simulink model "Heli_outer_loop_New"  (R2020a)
settings: Solver=FixedStepDiscrete  StartTime=0.0  StopTime=10.0  FixedStep=0.01  RelTol=1e-3  EnableMultiTasking=on
model workspace (MAT data in the model file):
  Ts : Simulink.Parameter (value not decoded)
symbols that are objects in the model workspace (value not decoded): Ts
undefined symbols (not defined in the file or in its folder): DiscIntNeverNeededParam
libraries: simulink x1

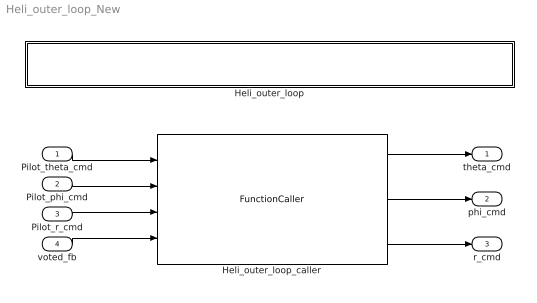
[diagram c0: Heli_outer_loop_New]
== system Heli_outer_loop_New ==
  Pilot_theta_cmd : Inport
  Pilot_phi_cmd : Inport  Port=2
  Pilot_r_cmd : Inport  Port=3
  voted_fb : Inport  Port=4
  Heli_outer_loop : Subsystem  TreatAsAtomicUnit=on
  Heli_outer_loop_caller : FunctionCaller  FunctionPrototype=[theta_cmd,phi_cmd,r_cmd] = Heli_outer_loop(Pilot_theta_cmd,Pilot_phi_cmd,Pilot_r_cmd,voted_fb)
  theta_cmd : Outport
  phi_cmd : Outport  Port=2
  r_cmd : Outport  Port=3
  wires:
  Pilot_theta_cmd/1 -> Heli_outer_loop_caller/1
  Pilot_phi_cmd/1 -> Heli_outer_loop_caller/2
  Pilot_r_cmd/1 -> Heli_outer_loop_caller/3
  voted_fb/1 -> Heli_outer_loop_caller/4
  Heli_outer_loop_caller/1 -> theta_cmd/1
  Heli_outer_loop_caller/2 -> phi_cmd/1
  Heli_outer_loop_caller/3 -> r_cmd/1

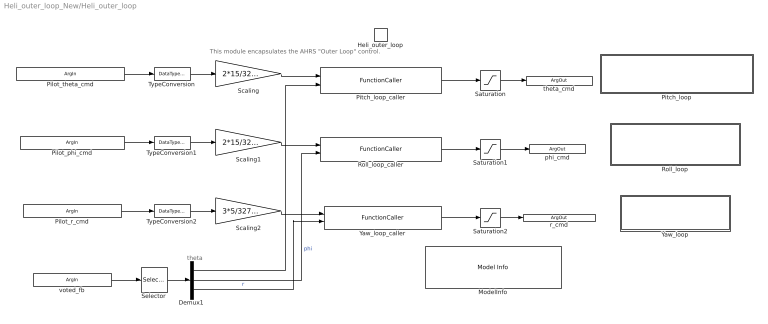
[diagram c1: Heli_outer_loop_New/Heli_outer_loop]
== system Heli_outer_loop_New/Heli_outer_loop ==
  note: theta
  note: This module encapsulates the AHRS "Outer Loop" control.
  Heli_outer_loop : TriggerPort  TriggerType=function-call  IsSimulinkFunction=on  FunctionName=Heli_outer_loop  FunctionVisibility=scoped  VariantControl=Variant  PortDimensions=1
  Demux1 : Demux  Outputs=3
  ModelInfo : simulink/Model-Wide Utilities/Model Info  Frame=on  DisplayStringWithTags=|  HorizontalTextAlignment=Center  LeftAlignmentValue=0.5
      | Model Name: %<ModelName>
      | Model Version: %<ModelVersion>
      | Last Modified: %<LastModificationDate>
      | 
      | Copyright 2016 The MathWorks, Inc.
  Pitch_loop : Subsystem  TreatAsAtomicUnit=on
  Pitch_loop_caller : FunctionCaller  FunctionPrototype=theta_cmd = Pitch_loop(Pilot_theta_cmd,theta)  InputArgumentSpecifications=double(1),double(1)  OutputArgumentSpecifications=double(1)
  Roll_loop : Subsystem  TreatAsAtomicUnit=on
  Roll_loop_caller : FunctionCaller  FunctionPrototype=phi_cmd = Roll_loop(Pilot_phi_cmd,phi)  InputArgumentSpecifications=double(1),double(1)  OutputArgumentSpecifications=double(1)
  Saturation : Saturate  UpperLimit=30  LowerLimit=-30
  Saturation1 : Saturate  UpperLimit=30  LowerLimit=-30
  Saturation2 : Saturate  UpperLimit=30  LowerLimit=-30
  Scaling : Gain  Gain=2*15/32767
  Scaling1 : Gain  Gain=2*15/32767
  Scaling2 : Gain  Gain=3*5/32767
  Selector : Selector  InputPortWidth=5  IndexOptions=Index vector (dialog)  Indices=[1 2 3]  OutputSizes=1
  TypeConversion : DataTypeConversion  OutDataTypeStr=double
  TypeConversion1 : DataTypeConversion  OutDataTypeStr=double
  TypeConversion2 : DataTypeConversion  OutDataTypeStr=double
  Yaw_loop : Subsystem  TreatAsAtomicUnit=on
  Yaw_loop_caller : FunctionCaller  FunctionPrototype=r_cmd = Yaw_loop(Pilot_r_cmd,r)  InputArgumentSpecifications=double(1), double(1)  OutputArgumentSpecifications=double(1)
  Pilot_theta_cmd : ArgIn  OutDataTypeStr=int16  ArgumentName=Pilot_theta_cmd
  Pilot_phi_cmd : ArgIn  Port=2  OutDataTypeStr=int16  ArgumentName=Pilot_phi_cmd
  Pilot_r_cmd : ArgIn  Port=3  OutDataTypeStr=int16  ArgumentName=Pilot_r_cmd
  voted_fb : ArgIn  Port=4  PortDimensions=5  ArgumentName=voted_fb
  theta_cmd : ArgOut  ArgumentName=theta_cmd
  phi_cmd : ArgOut  Port=2  ArgumentName=phi_cmd
  r_cmd : ArgOut  Port=3  ArgumentName=r_cmd
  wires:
  Selector/1 -> Demux1/1
  TypeConversion2/1 -> Scaling2/1
  Pilot_r_cmd/1 -> TypeConversion2/1
  Pilot_phi_cmd/1 -> TypeConversion1/1
  Saturation1/1 -> phi_cmd/1
  TypeConversion1/1 -> Scaling1/1
  Saturation2/1 -> r_cmd/1
  voted_fb/1 -> Selector/1
  Roll_loop_caller/1 -> Saturation1/1
  Yaw_loop_caller/1 -> Saturation2/1
  TypeConversion/1 -> Scaling/1
  Saturation/1 -> theta_cmd/1
  Pilot_theta_cmd/1 -> TypeConversion/1
  Scaling/1 -> Pitch_loop_caller/1
  Demux1/1 -> Pitch_loop_caller/2
  Scaling1/1 -> Roll_loop_caller/1
  Demux1/2 -> Roll_loop_caller/2  "phi"
  Pitch_loop_caller/1 -> Saturation/1
  Scaling2/1 -> Yaw_loop_caller/1
  Demux1/3 -> Yaw_loop_caller/2  "r"

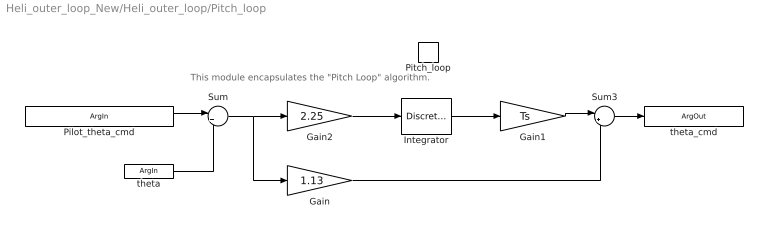
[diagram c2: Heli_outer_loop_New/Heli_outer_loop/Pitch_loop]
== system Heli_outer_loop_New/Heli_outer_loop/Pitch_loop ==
  note: This module encapsulates the "Pitch Loop" algorithm.
  Pitch_loop : TriggerPort  TriggerType=function-call  IsSimulinkFunction=on  FunctionName=Pitch_loop  FunctionVisibility=scoped  VariantControl=Variant  PortDimensions=1
  Gain : Gain  Gain=1.13
  Gain1 : Gain  Gain=Ts
  Gain2 : Gain  Gain=2.25
  Integrator : DiscreteIntegrator  IntegratorMethod=Accumulation: Forward Euler  SampleTime=-1  LimitOutput=on  UpperSaturationLimit=10  LowerSaturationLimit=-10  ICPrevOutput=DiscIntNeverNeededParam  ICPrevScaledInput=DiscIntNeverNeededParam
  Sum : Sum  Inputs=|+-  InputSameDT=on
  Sum3 : Sum  Inputs=|++
  Pilot_theta_cmd : ArgIn  ArgumentName=Pilot_theta_cmd
  theta : ArgIn  Port=2  ArgumentName=theta
  theta_cmd : ArgOut  ArgumentName=theta_cmd
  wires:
  Gain2/1 -> Integrator/1
  Sum3/1 -> theta_cmd/1
  Integrator/1 -> Gain1/1
  Gain/1 -> Sum3/2
  Gain1/1 -> Sum3/1
  Pilot_theta_cmd/1 -> Sum/1
  Sum/1 -> Gain/1, Gain2/1
  theta/1 -> Sum/2

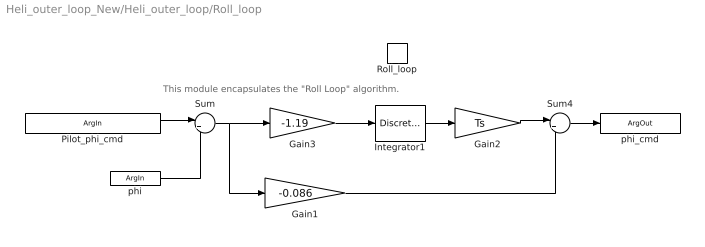
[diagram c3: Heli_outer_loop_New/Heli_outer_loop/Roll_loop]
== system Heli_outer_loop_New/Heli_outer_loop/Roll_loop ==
  note: This module encapsulates the "Roll Loop" algorithm.
  Roll_loop : TriggerPort  TriggerType=function-call  IsSimulinkFunction=on  FunctionName=Roll_loop  FunctionVisibility=scoped  VariantControl=Variant  PortDimensions=1
  Gain1 : Gain  Gain=-0.086
  Gain2 : Gain  Gain=Ts
  Gain3 : Gain  Gain=-1.19
  Integrator1 : DiscreteIntegrator  IntegratorMethod=Accumulation: Forward Euler  SampleTime=-1  LimitOutput=on  UpperSaturationLimit=10  LowerSaturationLimit=-10  ICPrevOutput=DiscIntNeverNeededParam  ICPrevScaledInput=DiscIntNeverNeededParam
  Sum : Sum  Inputs=|+-  InputSameDT=on
  Sum4 : Sum  Inputs=|++
  Pilot_phi_cmd : ArgIn  ArgumentName=Pilot_phi_cmd
  phi : ArgIn  Port=2  ArgumentName=phi
  phi_cmd : ArgOut  ArgumentName=phi_cmd
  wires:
  Sum4/1 -> phi_cmd/1
  Gain3/1 -> Integrator1/1
  Gain1/1 -> Sum4/2
  Integrator1/1 -> Gain2/1
  Gain2/1 -> Sum4/1
  phi/1 -> Sum/2
  Pilot_phi_cmd/1 -> Sum/1
  Sum/1 -> Gain1/1, Gain3/1

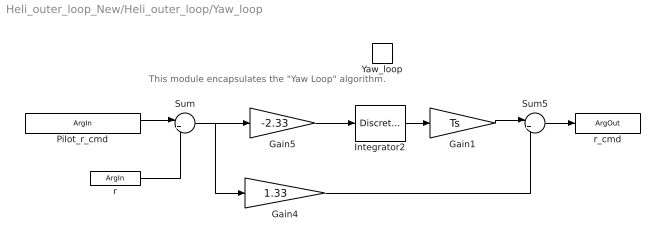
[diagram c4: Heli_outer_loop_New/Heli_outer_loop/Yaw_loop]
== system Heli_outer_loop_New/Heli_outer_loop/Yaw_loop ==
  note: This module encapsulates the "Yaw Loop" algorithm.
  Yaw_loop : TriggerPort  TriggerType=function-call  IsSimulinkFunction=on  FunctionName=Yaw_loop  FunctionVisibility=scoped  VariantControl=Variant  PortDimensions=1
  Gain1 : Gain  Gain=Ts
  Gain4 : Gain  Gain=1.33
  Gain5 : Gain  Gain=-2.33
  Integrator2 : DiscreteIntegrator  IntegratorMethod=Accumulation: Forward Euler  SampleTime=-1  LimitOutput=on  UpperSaturationLimit=10  LowerSaturationLimit=-10  ICPrevOutput=DiscIntNeverNeededParam  ICPrevScaledInput=DiscIntNeverNeededParam
  Sum : Sum  Inputs=|+-  InputSameDT=on
  Sum5 : Sum  Inputs=|++
  Pilot_r_cmd : ArgIn  ArgumentName=Pilot_r_cmd
  r : ArgIn  Port=2  ArgumentName=r
  r_cmd : ArgOut  ArgumentName=r_cmd
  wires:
  Integrator2/1 -> Gain1/1
  Gain4/1 -> Sum5/2
  Gain5/1 -> Integrator2/1
  Sum5/1 -> r_cmd/1
  Gain1/1 -> Sum5/1
  r/1 -> Sum/2
  Pilot_r_cmd/1 -> Sum/1
  Sum/1 -> Gain4/1, Gain5/1
